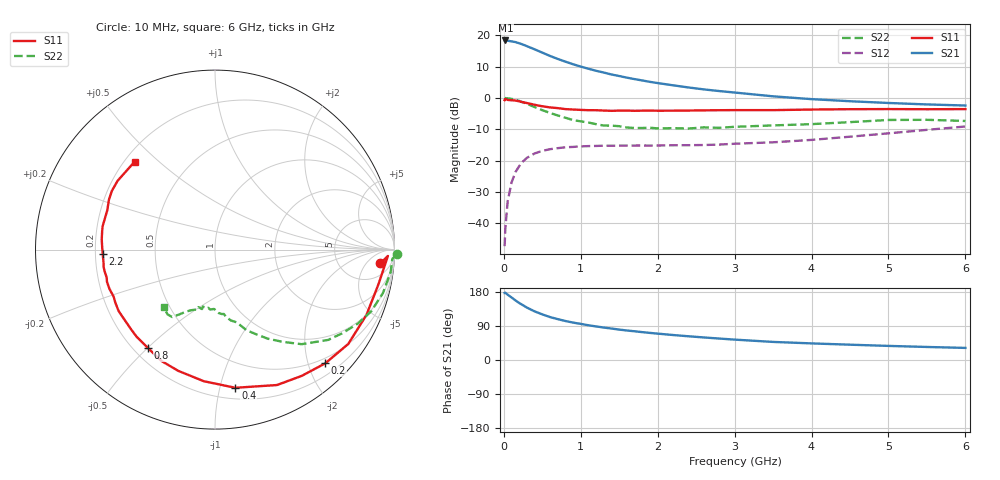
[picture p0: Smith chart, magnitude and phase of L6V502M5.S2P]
!  INFINEON TECHNOLOGIES Small Signal Semiconductors
! BFR380L3 , Si-NPN RF-Transistor in TSLP-3-1
!  Vce=0.5 V,  Ic=2.5 mA
! Common Emitter S-Parameters:  07. March 2005
#  GHz  S  MA  R  50
! f  S11  S21  S12  S22
! GHz  Mag  Ang  Mag  Ang  Mag  Ang  Mag  Ang
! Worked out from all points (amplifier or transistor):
!   36 points, 10 MHz to 6 GHz, reference 50 ohm
!   highest |S21| = 18.4 dB at 20 MHz (marker M1)
!   |S21| within 3 dB of that: start of sweep to 415.6 MHz
!   unconditionally stable (mu >= 1): 2.529 GHz to 5.075 GHz
!   at 250 MHz: K = 0.11, MSG = 18.6 dB, |S12| = -20.2 dB
!   at 1.4 GHz: K = 0.64, MSG = 11.4 dB, |S12| = -15.3 dB
!   at 6 GHz: K = 0.98, MSG = 3.3 dB, |S12| = -9.1 dB
!   S11 on the Smith chart (normalised r, x): 10 MHz: 12, -13; 200 MHz: 0.40, -2.30; 400 MHz: 0.29, -1.12; 800 MHz: 0.26, -0.50; 2.2 GHz: 0.23, -0.02; 6 GHz: 0.24, +0.42
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0.01  0.9241 -4.8  8.227 176.9  0.0043 87.6  1.012 -1.5
0.02  0.9641 -2.1  8.275 177.4  0.0085 91.6  0.9891 -3.0
0.05  0.9309 -12.0  8.19 172.3  0.0224 84.1  0.9866 -7.3
0.1  0.919 -23.3  8.009 165.0  0.0447 77.2  0.9665 -14.5
0.15  0.9098 -35.3  7.799 157.5  0.0651 70.3  0.9357 -21.6
0.2  0.8826 -45.9  7.459 150.4  0.0816 65.2  0.896 -27.4
0.25  0.8535 -55.5  7.101 144.4  0.0972 60.0  0.8479 -33.4
0.3  0.8299 -65.4  6.703 138.3  0.1106 55.4  0.8066 -38.6
0.4  0.7782 -81.6  5.971 128.3  0.1299 47.6  0.7148 -47.5
0.5  0.7361 -94.8  5.286 120.4  0.1429 42.2  0.6379 -53.7
0.6  0.7059 -106.9  4.684 113.3  0.152 37.6  0.5766 -59.4
0.8  0.6636 -124.1  3.8 102.9  0.163 32.1  0.4827 -68.6
0.9  0.6531 -131.9  3.449 98.7  0.1653 30.3  0.4432 -71.6
1.1  0.6376 -142.6  2.923 91.6  0.1703 28.0  0.4051 -77.3
1.3  0.629 -152.0  2.541 85.6  0.173 26.8  0.3619 -82.2
1.6  0.6281 -163.3  2.108 77.8  0.1737 26.5  0.3373 -89.6
2.2  0.6262 -177.7  1.591 65.9  0.1756 29.9  0.3295 -97.2
2.8  0.637 170.8  1.288 56.6  0.1801 36.0  0.3332 -106.1
3.5  0.6388 160.0  1.061 47.7  0.1957 42.8  0.3642 -111.8
4.5  0.6612 150.4  0.886 40.4  0.2406 52.7  0.411 -118.7
5.5  0.6603 138.9  0.788 34.4  0.3094 56.3  0.4475 -126.3
6  0.6636 132.4  0.757 31.9  0.3501 56.1  0.4288 -131.7
